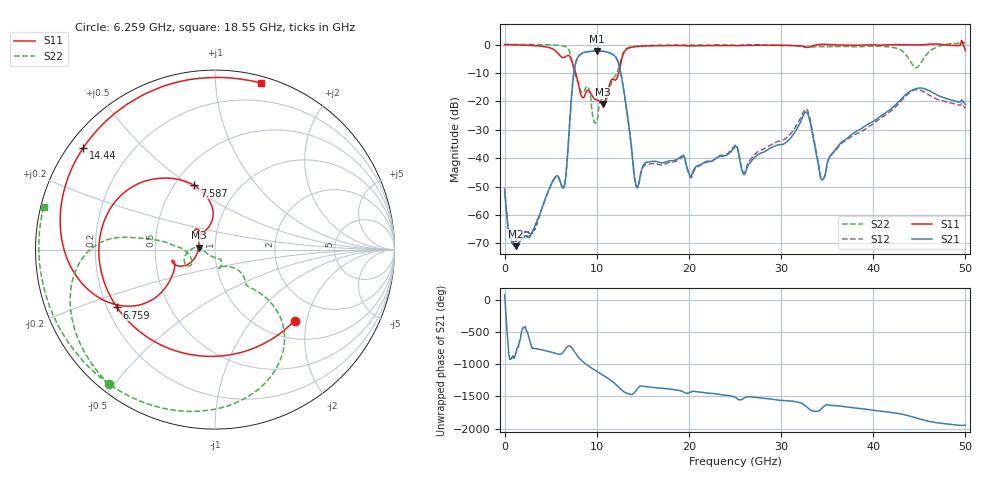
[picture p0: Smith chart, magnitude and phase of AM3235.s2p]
!Agilent Technologies,E8364B,MY43040894,A.07.50.67
!Agilent E8364B: A.07.50.67
!Date: Tuesday, May 02, 2023 05:37:30
!Correction: S11(Full 2 Port(1,2))
!S21(Full 2 Port(1,2))
!S12(Full 2 Port(1,2))
!S22(Full 2 Port(1,2))
!S2P File: Measurements: S11, S21, S12, S22:
# Hz S  dB  R 50
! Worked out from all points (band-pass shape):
!   6401 points, 10 MHz to 50 GHz, reference 50 ohm
!   highest |S21| = -2.20 dB at 10.03 GHz (marker M1); lowest = -70.9 dB at 1.236 GHz (marker M2)
!   |S21| within 3 dB of the highest: 7.84 GHz to 12.21 GHz (4.367 GHz wide, 43.6 % of centre)
!   lowest |S11| = -20.9 dB at 10.66 GHz (marker M3), VSWR 1.20, Z = 41.8 + j0.939 ohm
!   |S11| at or under -10 dB: 7.723 GHz to 12.39 GHz (4.668 GHz wide, 46.4 % of centre)
!   |S22| runs from -27.6 to 0.6 dB; largest |S21 - S12| = 0.029
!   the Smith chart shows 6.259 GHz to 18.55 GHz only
!   S11 on the Smith chart (normalised r, x): 6.259 GHz: 1.39, -1.70; 6.759 GHz: 0.24, -0.26; 7.587 GHz: 0.63, +0.52; 14.44 GHz: 0.04, +0.34; 18.55 GHz: 0.05, +1.31
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1e7  -0.02 -7.2  -51.99 85.3  -50.54 106.1  0.03 -1.6
1.236317e9  -0.06 -82.9  -70.94 -98.0  -68.93 -5.8  0.03 -19.9
3.142186e9  -0.35 -169.1  -65.09 -30.5  -65.37 177.1  0.02 -52.5
5.102731e9  -1.35 107.4  -48.84 -90.5  -49.12 -91.7  -0.09 -93.2
6.25875e9  -4.52 -41.8  -49.99 -107.2  -50.16 -106.5  -0.41 -128.0
6.75865e9  -3.96 -149.5  -42.31 -12.8  -42.46 -11.7  -1.00 -152.5
7.586609e9  -8.50 107.9  -8.61 -85.1  -8.69 -84.8  -9.39 170.7
8.34427e9  -18.10 109.8  -3.19 140.5  -3.23 140.6  -16.69 -167.6
1.003143e10  -19.52 147.1  -2.20 -31.7  -2.24 -32.0  -26.75 -84.5
1.066412e10  -20.87 172.9  -2.32 -87.7  -2.35 -88.0  -19.56 -77.6
1.21482e10  -12.10 -155.5  -4.83 116.6  -4.84 115.3  -10.29 -45.9
1.444461e10  -0.65 142.5  -49.97 63.9  -50.40 64.6  -0.46 -122.3
1.667854e10  -0.39 101.6  -41.31 70.1  -42.17 72.6  -0.21 -166.3
1.855317e10  -0.33 74.7  -40.63 42.6  -41.12 45.5  -0.14 166.0
2.5005e10  -0.34 -6.8  -35.91 -72.5  -35.38 -66.1  -0.15 91.1
3.333927e10  -0.55 -109.2  -30.27 78.4  -29.25 69.5  -0.82 -18.6
3.453434e10  0.09 -126.4  -47.56 130.3  -47.25 116.0  -0.70 -41.6
3.772902e10  -0.22 -160.3  -31.45 126.8  -32.19 118.6  -0.75 -108.7
4.167354e10  -0.09 166.7  -23.26 55.1  -23.96 53.0  -0.77 165.0
4.454797e10  -0.11 144.7  -15.61 -29.9  -15.92 -35.0  -8.07 3.3
4.582896e10  0.04 135.0  -15.85 -80.6  -17.26 -86.0  -3.32 -122.7
5e10  -2.15 164.3  -21.07 -147.7  -22.39 -149.1  0.65 152.4
